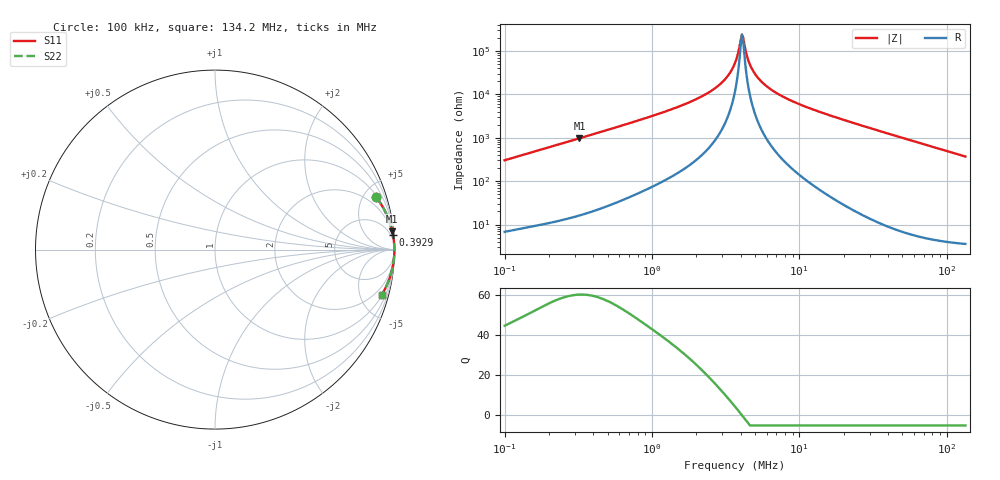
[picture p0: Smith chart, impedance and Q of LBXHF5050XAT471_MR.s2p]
! LBXHF5050XAT471_MR  S-PARAMETER MODEL  ( General Type )
! Model Generated by TAIYO YUDEN Corporation (http://www.ty-top.com)
! Version 1.0
! TAIYO YUDEN Control No. 200511NI43SB-FBB
! Copyright(c) 2020 TAIYO YUDEN CO.,LTD. All Rights Reserved.
! Product Description (link to TY-COMPAS)
! https://ds.yuden.co.jp/TYCOMPAS/or/detail?pn=LBXHF5050XAT471MMR&u=M
! Products Name : Inductors
! Characteristics :
!  Inductance : 470 uH , SRF(min) : 2.5 MHz , DC Resistance(max) : 3.672 Ohm
!  Rated Current : Saturation :250 mA , Temp Rise : 170 mA
!  Case Size : 5.0 x 5.0 / 0.197 x 0.197 [mm/inch] , Thickness : 3.1 / 0.122 [mm/inch]
!  (Conditions: Temperature = 25 degC , DC Bias Current/Voltage = 0A / 0V)
! External Node Assignments :
!  1  o---GGG---o  2
! GND o---------o GND
! Frequency Range : 0.1MHz  -  134.160692MHz  [ 402 STEP ]
# MHz S RI R 50
! Freq[MHz].  S11 Real  S11 Imag  S21 Real  S21 Imag  S12 Real  S12 Imag  S22 Real  S22 Imag
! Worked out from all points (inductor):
!   401 points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, 100 kHz to 134.2 MHz, reference 50 ohm
!   read as one part in series: L = 480 uH near 103.7 kHz
!   highest Q = 60.2 at 322.3 kHz (marker M1), where L = 480 uH
!   self-resonance near 4.081 MHz
!   S11 on the Smith chart (normalised r, x): 100 kHz: 1.14, +6.06; 392.9 kHz: 1, +24; 134.2 MHz: 1.07, -7.39
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0.1  0.8964 0.2937  0.1036 -0.2937  0.1036 -0.2937  0.8964 0.2937
0.322284  0.9879 0.1014  0.0121 -0.1014  0.0121 -0.1014  0.9879 0.1014
0.334101  0.9887 0.0979  0.0113 -0.0979  0.0113 -0.0979  0.9887 0.0979
0.39287  0.9916 0.0833  0.00841 -0.0833  0.00841 -0.0833  0.9916 0.0833
1.116232  0.9985 0.0278  0.00146 -0.0278  0.00146 -0.0278  0.9985 0.0278
1.881513  0.9993 0.0141  0.000722 -0.0141  0.000722 -0.0141  0.9993 0.0141
2.648924  0.9995 0.00741  0.000511 -0.00741  0.000511 -0.00741  0.9995 0.00741
3.287746  0.9996 0.00365  0.000443 -0.00365  0.000443 -0.00365  0.9996 0.00365
3.533251  0.9996 0.00244  0.000428 -0.00244  0.000428 -0.00244  0.9996 0.00244
3.729338  0.9996 0.00155  0.00042 -0.00155  0.00042 -0.00155  0.9996 0.00155
4.007818  0.9996 0.000357  0.000412 -0.000357  0.000412 -0.000357  0.9996 0.000357
4.080628  0.9996 5.95e-05  0.000411 -5.95e-05  0.000411 -5.95e-05  0.9996 5.95e-05
4.154761  0.9996 -0.000238  0.00041 0.000238  0.00041 0.000238  0.9996 -0.000238
4.230241  0.9996 -0.000535  0.000409 0.000535  0.000409 0.000535  0.9996 -0.000535
4.465009  0.9996 -0.00143  0.000408 0.00143  0.000408 0.00143  0.9996 -0.00143
4.712806  0.9996 -0.00233  0.000408 0.00233  0.000408 0.00233  0.9996 -0.00233
5.064724  0.9996 -0.00353  0.000412 0.00353  0.000412 0.00353  0.9996 -0.00353
5.541803  0.9996 -0.00507  0.000422 0.00507  0.000422 0.00507  0.9996 -0.00507
7.52619  0.9995 -0.0107  0.000506 0.0107  0.000506 0.0107  0.9995 -0.0107
12.23742  0.9991 -0.0219  0.000878 0.0219  0.000878 0.0219  0.9991 -0.0219
40.88529  0.9928 -0.081  0.00719 0.081  0.00719 0.081  0.9928 -0.081
134.1607  0.9297 -0.2508  0.0703 0.2508  0.0703 0.2508  0.9297 -0.2508
